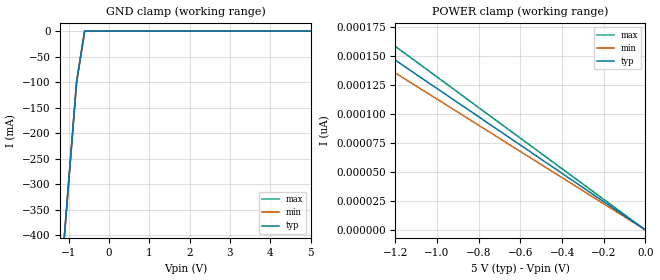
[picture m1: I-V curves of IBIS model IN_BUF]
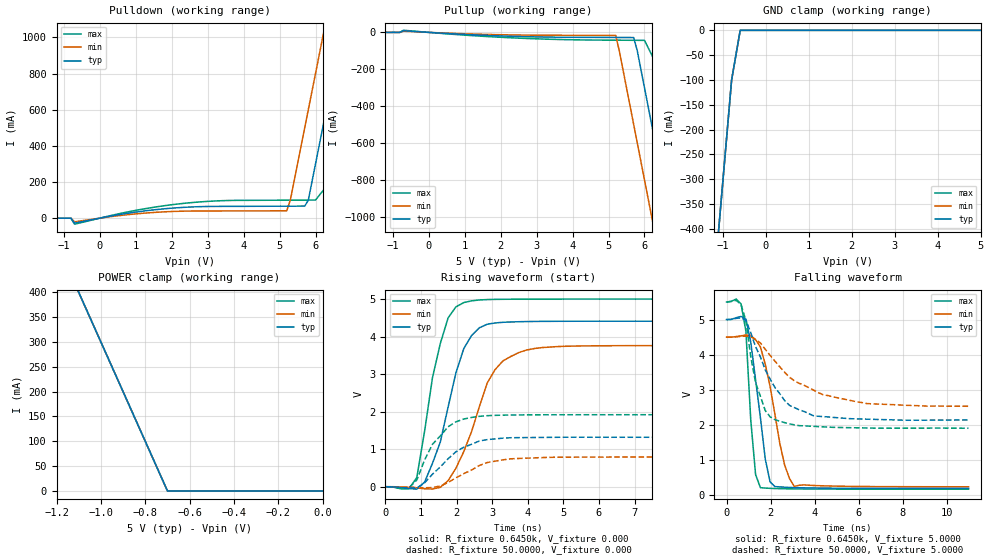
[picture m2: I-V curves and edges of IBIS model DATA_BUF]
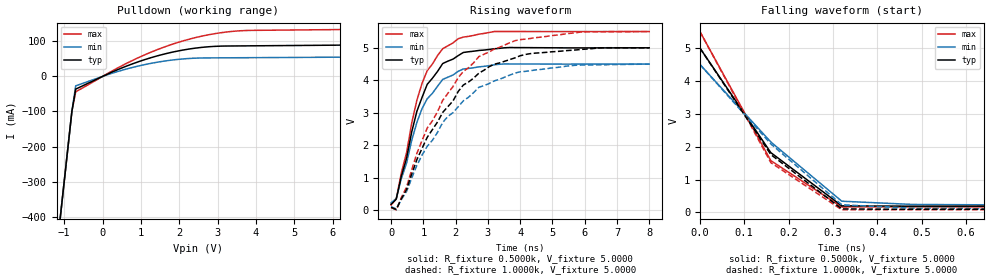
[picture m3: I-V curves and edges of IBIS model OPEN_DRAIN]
| IBIS file m48t18.ibs created by s2ibis2 version 1.1
| North Carolina State University Electronics Research Laboratory  1995
[IBIS ver]   2.1
[File name]   m48t18_pdip28.ibs
[File Rev]   4.0
[Date]   September 12, 2001
[Source]   ST models
[Notes]   Extracted view used. Simulation with Eldo (the s2ibis2 code
   was slightly changed to run with Eldo)
[Disclaimer] We used the packaging information of the T212. It should be
   the same but need to be confirme. We also put a 1.0 ohm
   resistor in series with the output and input for current
   limitation.
[Copyright]   ST Microelectronics Inc.
|   Component m48t18
[Component]   m48t18
[Manufacturer]   ST Microelectronics [Package]
[Package]
| variable   typ   min   max
R_pkg   2.0000m   2.0000m   2.0000m
L_pkg   9.5000nH   4.2000nH   14.8000nH
C_pkg   2.1000pF   1.4000pF   2.9000pF
[Pin]  signal_name   model_name   R_pin   L_pin   C_pin
| gdb  dummy   dummy
| od   dummy   dummy
| pd   dummy   dummy
1   INT#   OPEN_DRAIN
2   A12   IN_BUF
3   A7   IN_BUF
4   A6   IN_BUF
5   A5   IN_BUF
6   A4   IN_BUF
7   A3   IN_BUF
8   A2   IN_BUF
9   A1   IN_BUF
10   A0   IN_BUF
11   DQ0   DATA_BUF
12   DQ1   DATA_BUF
13   DQ2   DATA_BUF
14   VSS   GND
15   DQ3   DATA_BUF
16   DQ4   DATA_BUF
17   DQ5   DATA_BUF
18   DQ6   DATA_BUF
19   DQ7   DATA_BUF
20   E1#   IN_BUF
21   A10   IN_BUF
22   G#   IN_BUF
23   A11   IN_BUF
24   A9   IN_BUF
25   A8   IN_BUF
26   E2   IN_BUF
27   W#   IN_BUF
28   VCC   POWER
| Models and submodels in the file (3): IN_BUF (Input), DATA_BUF (I/O), OPEN_DRAIN (Open_drain)
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|   Model IN_BUF
[Model]   IN_BUF
Model_type   Input
Vinl =   0.8000V
Vinh =   2.2000V
C_comp   2.0100pF   1.9700pF   2.0600pF
[Temperature Range]   27.0000   70.0000   0.000
[Voltage Range]   5.0000V   4.5000V   5.5000V
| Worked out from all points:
|   GND clamp passes 1 mA (typ) near -0.60 V on its own axis
[GND_clamp]
| voltage   I(typ)   I(min)   I(max)
-5V       -4.3A      -4.3A      -4.3A
-1.2V     -500mA     -500mA     -500mA
-1V       -300mA     -300mA     -300mA
-800mV    -100mA     -100mA     -100mA
-600mV    -2.424uA   -939.7nA   -1.758uA
5V        2.595nA    12.1pA     3.525nA
[POWER_clamp]
| voltage   I(typ)   I(min)   I(max)
-5V       610.7pA    564.8pA    660.3pA
-1.6V     195.4pA    180.7pA    211.3pA
-1.5V     183.2pA    169.4pA    198.1pA
-1.4V     171pA      158.1pA    184.9pA
-1.3V     158.8pA    146.8pA    171.7pA
0V        0A         0A         0A
|   Model DATA_BUF
[Model]   DATA_BUF
Model_type   I/O
Polarity   Inverting
Enable   Active-High
Vinl =   0.8000V
Vinh =   2.2000V
Vmeas =   1.5000V
Cref =1.000e-10F
Rref =   0.6420k
Vref =   1.7500V
C_comp   4.3700pF   4.2600pF   4.4800pF
[Temperature Range]   27.0000   70.0000   0.000
[Voltage Range]   5.0000V   4.5000V   5.5000V
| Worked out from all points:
|   slope of the pulldown table from 0 to 0.75 V, typ, clamps not added: 28.6 ohm
|   slope of the pullup table from 0 to 0.75 V, typ, clamps not added: 87.2 ohm
|   GND clamp passes 1 mA (typ) near -0.60 V on its own axis
|   POWER clamp passes 1 mA (typ) near -0.70 V on its own axis
|   rising waveform, R_fixture 0.6450k, V_fixture 0.000: 20-80 % time 728ps typ, 902ps min, 586ps max; typ from 0 V to 4.42 V
|   rising waveform, R_fixture 50.0000, V_fixture 0.000: 20-80 % time 949ps typ, 986ps min, 739ps max; typ from 0 V to 1.32 V
|   falling waveform, R_fixture 0.6450k, V_fixture 5.0000: 20-80 % time 570ps typ, 770ps min, 328ps max; typ from 5 V to 0.195 V
|   falling waveform, R_fixture 50.0000, V_fixture 5.0000: 20-80 % time 1.41ns typ, 2.33ns min, 722ps max; typ from 5 V to 2.14 V
[Pulldown]
| voltage   I(typ)   I(min)   I(max)
-5V       0A         0A         0A
-700mV    -27.18mA   -20.3mA    -33.2mA
2.2V      58.09mA    38.12mA    78.91mA
5.2V      66.27mA    40.69mA    99.49mA
5.7V      66.6mA     500mA      99.87mA
5.8V      100mA      600mA      99.95mA
6V        300mA      800mA      100.1mA
6.4V      700mA      1.2A       200mA
6.8V      1.1A       1.6A       600mA
7.2V      1.5A       2A         1A
7.6V      1.9A       2.4A       1.4A
10V       4.3A       4.8A       3.8A
[Pullup]
| voltage   I(typ)   I(min)   I(max)
-5V       0A         0A         0A
-700mV    8.869mA    6.357mA    11.51mA
2.3V      -21.18mA   -13.79mA   -29.47mA
5.2V      -27.66mA   -16.47mA   -42.41mA
5.7V      -28.2mA    -500mA     -43.01mA
5.8V      -100mA     -600mA     -43.12mA
6V        -300mA     -800mA     -43.36mA
6.4V      -700mA     -1.2A      -200mA
6.8V      -1.1A      -1.6A      -600mA
7.2V      -1.5A      -2A        -1A
7.6V      -1.9A      -2.4A      -1.4A
10V       -4.3A      -4.8A      -3.8A
[GND_clamp]
| voltage   I(typ)   I(min)   I(max)
-5V       -4.3A      -4.3A      -4.3A
-1.2V     -500mA     -500mA     -500mA
-1V       -300mA     -300mA     -300mA
-800mV    -100mA     -100mA     -100mA
-600mV    -26.04uA   -10.29uA   -17.63uA
5V        60.14pA    77.13nA    9.57nA
[POWER_clamp]
| voltage   I(typ)   I(min)   I(max)
-5V       4.3A       4.3A       4.3A
-1.1V     400mA      400mA      400mA
-1V       300mA      300mA      300mA
-700mV    12.45uA    2.467uA    49.04uA
0V        0A         0A         0A
[Ramp]
| variable   typ   min   max
dV/dt_r   2.6479/0.6792n   2.2570/0.9892n   3.0025/0.5069n
dV/dt_f   2.8823/0.4818n   2.5551/0.7573n   3.1961/0.3269n
R_load = 0.6420k
[Rising Waveform]
R_fixture = 0.6450k
V_fixture = 0.000
V_fixture_min = 0.000
V_fixture_max = 0.000
| time   V(typ)   V(min)   V(max)
0s        1.435nV    1.811nV    1.234nV
660ps     -49.1mV    -16.03mV   -55.25mV
880ps     -65.18mV   -29.56mV   245.1mV
1.32ns    623.6mV    -60.7mV    2.907V
1.54ns    1.19V      -16.59mV   3.818V
1.76ns    2.127V     162.1mV    4.505V
2.2ns     3.683V     937mV      4.913V
2.86ns    4.336V     2.77V      4.993V
3.74ns    4.402V     3.577V     5.003V
11ns      4.416V     3.765V     5.006V
[Rising Waveform]
R_fixture = 50.0000
V_fixture = 0.000
V_fixture_min = 0.000
V_fixture_max = 0.000
| time   V(typ)   V(min)   V(max)
0s        988.3pV    1.126nV    903.7pV
660ps     -34.03mV   -11.46mV   -26.74mV
880ps     -35.92mV   -19.64mV   177.9mV
1.1ns     104.7mV    -29.66mV   715.2mV
1.32ns    333.2mV    -19.76mV   1.133V
1.76ns    746.2mV    113.1mV    1.599V
2.42ns    1.133V     446.3mV    1.849V
2.86ns    1.257V     645.7mV    1.895V
3.74ns    1.309V     753.5mV    1.915V
11ns      1.32V      791.9mV    1.921V
[Falling Waveform]
R_fixture = 0.6450k
V_fixture = 5.0000
V_fixture_min = 4.5000
V_fixture_max = 5.5000
| time   V(typ)   V(min)   V(max)
0s        5V         4.5V       5.5V
660ps     5.089V     4.537V     5.447V
880ps     5.012V     4.559V     4.668V
1.1ns     4.363V     4.549V     2.147V
1.32ns    3.288V     4.428V     588.3mV
1.54ns    2.209V     4.221V     214.9mV
1.98ns    379mV      3.094V     195.8mV
2.64ns    228mV      862.7mV    184mV
3.08ns    216.5mV    248.5mV    179.8mV
11ns      195.2mV    240.4mV    172.3mV
[Falling Waveform]
R_fixture = 50.0000
V_fixture = 5.0000
V_fixture_min = 4.5000
V_fixture_max = 5.5000
| time   V(typ)   V(min)   V(max)
0s        5V         4.5V       5.5V
660ps     5.048V     4.522V     5.426V
880ps     4.981V     4.53V      4.971V
1.32ns    4.226V     4.431V     3.206V
1.76ns    3.57V      4.156V     2.411V
2.2ns     3.066V     3.817V     2.152V
2.86ns    2.558V     3.358V     2.032V
4.4ns     2.237V     2.857V     1.946V
6.38ns    2.165V     2.609V     1.914V
11ns      2.143V     2.532V     1.906V
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|   Model OPEN_DRAIN
[Model]   OPEN_DRAIN
Model_type   Open_drain
Polarity   Inverting
C_comp   2.9700pF   2.9100pF   3.0000pF
[Temperature Range]   27.0000   70.0000   0.000
[Voltage Range]   5.0000V   4.5000V   5.5000V
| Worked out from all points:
|   slope of the pulldown table from 0 to 0.75 V, typ, clamps not added: 21.7 ohm
|   rising waveform, R_fixture 0.5000k, V_fixture 5.0000: 20-80 % time 912ps typ, 961ps min, 889ps max; typ from 0.191 V to 5 V
|   rising waveform, R_fixture 1.0000k, V_fixture 5.0000: 20-80 % time 1.87ns typ, 1.92ns min, 1.82ns max; typ from 0.096 V to 5 V
|   falling waveform, R_fixture 0.5000k, V_fixture 5.0000: 20-80 % time 177ps typ, 196ps min, 155ps max; typ from 5 V to 0.19 V
|   falling waveform, R_fixture 1.0000k, V_fixture 5.0000: 20-80 % time 178ps typ, 196ps min, 155ps max; typ from 5 V to 0.095 V
[Pulldown]
| voltage   I(typ)   I(min)   I(max)
-5V       -4.3A      -4.3A      -4.3A
-1.4V     -700mA     -700mA     -700mA
-1V       -300mA     -300mA     -300mA
-800mV    -100mA     -100mA     -100mA
-700mV    -36.17mA   -26.91mA   -43.89mA
600mV     28.37mA    20.4mA     35.85mA
1.3V      54.61mA    38.06mA    70.79mA
2V        73.23mA    48.91mA    98.07mA
2.7V      83.97mA    52.75mA    117.4mA
3.4V      86.82mA    53.16mA    128.6mA
3.9V      87.24mA    53.46mA    131.3mA
10V       92.87mA    58.03mA    137.9mA
[Ramp]
| variable   typ   min   max
dV/dt_r   2.9103/1.2008n   2.5893/1.2060n   3.2198/1.1564n
dV/dt_f   2.9109/-81.9817 p   2.5907/0.1250n   3.2203/84.3654p
R_load = 0.6420k
[Rising Waveform]
R_fixture = 0.5000k
V_fixture = 5.0000
V_fixture_min = 4.5000
V_fixture_max = 5.5000
| time   V(typ)   V(min)   V(max)
0s        191.2mV    234.1mV    169.3mV
160ps     350.1mV    367mV      357.6mV
480ps     1.607V     1.455V     1.776V
640ps     2.417V     2.158V     2.691V
960ps     3.478V     3.133V     3.909V
1.12ns    3.878V     3.434V     4.299V
1.6ns     4.517V     4.029V     4.973V
2.24ns    4.857V     4.349V     5.329V
3.2ns     4.971V     4.478V     5.502V
8ns       5.001V     4.5V       5.5V
[Rising Waveform]
R_fixture = 1.0000k
V_fixture = 5.0000
V_fixture_min = 4.5000
V_fixture_max = 5.5000
| time   V(typ)   V(min)   V(max)
0s        96.13mV    117.8mV    85.18mV
160ps     28.45mV    47.67mV    22.14mV
480ps     646.4mV    585.2mV    720.9mV
800ps     1.566V     1.389V     1.758V
1.12ns    2.25V      1.974V     2.533V
1.6ns     3.015V     2.707V     3.389V
2.24ns    3.858V     3.371V     4.274V
2.72ns    4.22V      3.788V     4.73V
4.32ns    4.822V     4.296V     5.288V
8ns       5.001V     4.499V     5.5V
[Falling Waveform]
R_fixture = 0.5000k
V_fixture = 5.0000
V_fixture_min = 4.5000
V_fixture_max = 5.5000
| time   V(typ)   V(min)   V(max)
0s        5V         4.5V       5.5V
160ps     1.818V     2.142V     1.574V
320ps     200.5mV    341.5mV    166mV
480ps     190.5mV    243.1mV    169.9mV
640ps     191.4mV    232.1mV    169.5mV
8ns       190.4mV    233.5mV    169.9mV
[Falling Waveform]
R_fixture = 1.0000k
V_fixture = 5.0000
V_fixture_min = 4.5000
V_fixture_max = 5.5000
| time   V(typ)   V(min)   V(max)
0s        5V         4.5V       5.5V
160ps     1.759V     2.083V     1.514V
320ps     107.8mV    233.6mV    81.94mV
480ps     95.33mV    129.3mV    85.64mV
640ps     96.42mV    115.3mV    85.32mV
8ns       95.33mV    117.1mV    85.69mV
